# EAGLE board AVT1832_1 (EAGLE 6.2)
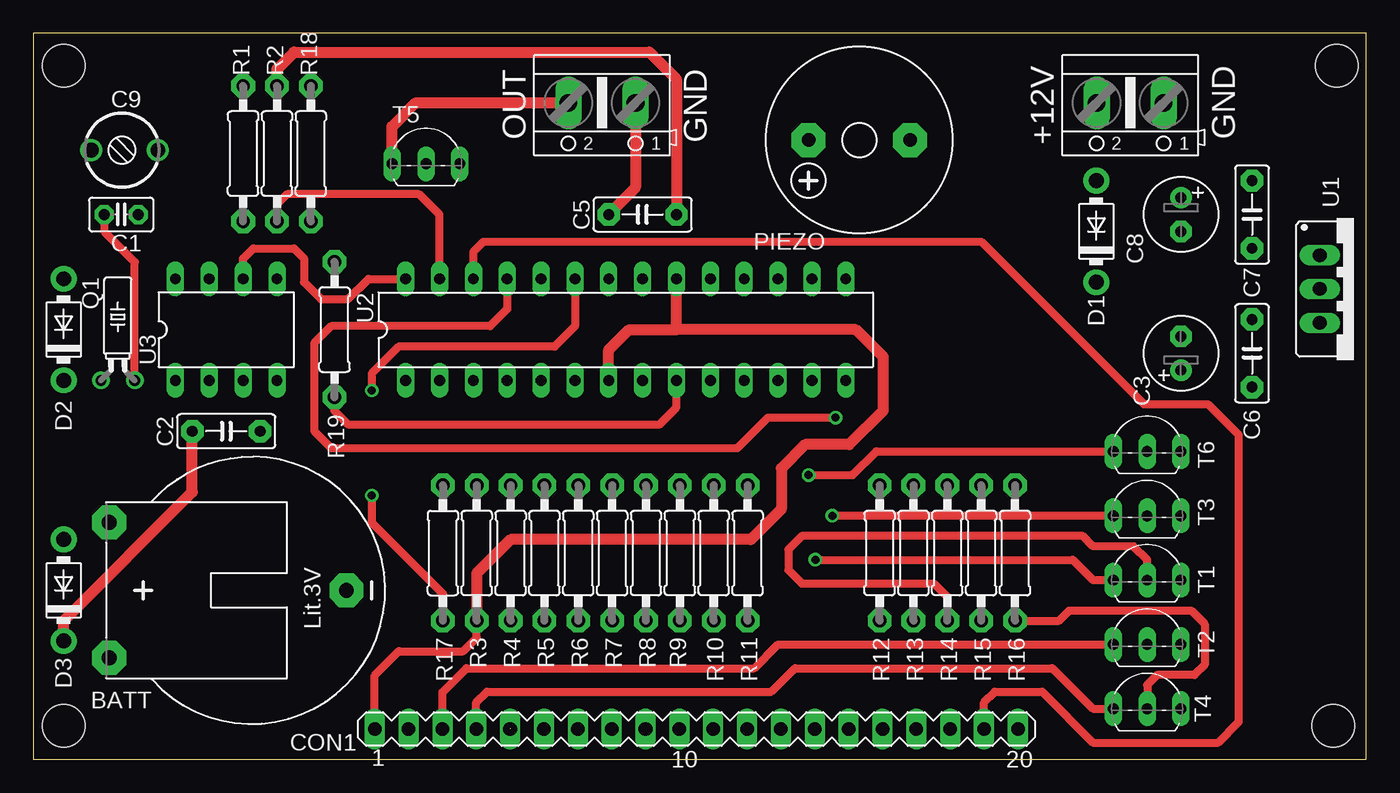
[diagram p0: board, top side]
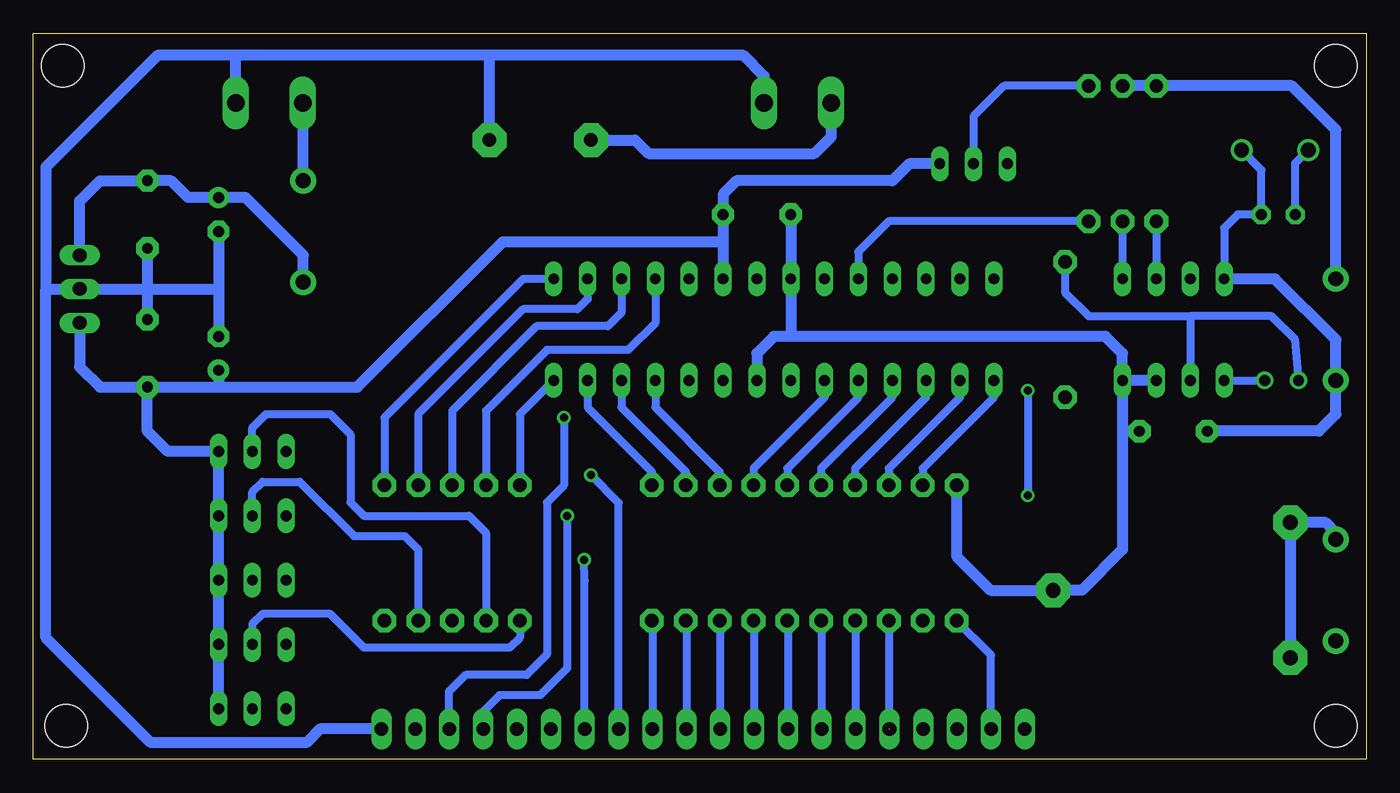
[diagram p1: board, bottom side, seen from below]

Size 99.99 x 54.49 mm. Coordinates in mm from the lower left corner, seen from the top.
Outline: 99.99,0 99.99,54.49 0,54.49 0,0 99.99,0
Copper layers (1*16): Top 0.035mm / dielectric 1.5mm / Bottom 0.035mm
Design rules: minimum track width 10mil, minimum drill 24mil, track to track 8mil, track to pad 8mil, pad to pad 8mil, via to via 8mil, smd to smd 8mil, copper to edge 40mil, drill to drill 8mil, minimum pad ring 10mil, minimum via ring 8mil, stop-mask expansion 4mil, vias tented up to drill 0mil, thermal gap 10mil
Holes 3.2 mm at 97.78,52.07 2.28,52.07 97.53,2.54 2.28,2.54

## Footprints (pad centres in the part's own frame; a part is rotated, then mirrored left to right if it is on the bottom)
AK500/2 = drill 1.321 long: 1 -2.515,0; 2 2.515,0
CR2032H = drill 1.118 pad 2.54 octagon: + 5.08,10.795; +@1 -5.08,10.795; - 0,-6.985
C025-025X050 = drill 0.813 pad 1.422 octagon: 1 -1.27,0; 2 1.27,0
C050-025X075 = drill 0.813 pad 1.676 octagon: 1 -2.54,0; 2 2.54,0
E2,5-6 = drill 0.813 pad 1.6: + -1.27,0 | drill 0.813 pad 1.6 octagon: - 1.27,0
CTRIM3050.504 = drill 1.1: 1 -2.5,0; 2 2.5,0
MA20-1 = drill 1.016 long: 1 -24.13,0; 2 -21.59,0; 3 -19.05,0; 4 -16.51,0; 5 -13.97,0; 6 -11.43,0; 7 -8.89,0; 8 -6.35,0; 9 -3.81,0; 10 -1.27,0; 11 1.27,0; 12 3.81,0; 13 6.35,0; 14 8.89,0; 15 11.43,0; 16 13.97,0; 17 16.51,0; 18 19.05,0; 19 21.59,0; 20 24.13,0
DO41-10 = drill 1.118 pad 1.93: A 3.81,0; C -3.81,0
F/CM12P = drill 1.016 pad 2.54 octagon: + 3.81,0; - -3.81,0
TC26H = drill 0.813: 1 -1.27,0; 2 1.27,0
0207/10 = drill 1 pad 1.778 octagon: 1 -5.08,0; 2 5.08,0
TO92-EBC = drill 0.813 long: B 0,-1.27; C -2.54,-1.27; E 2.54,-1.27
78XXS = drill 1.016 long: GND 0,-2.54; IN -2.54,-2.54; OUT 2.54,-2.54
DIL28-3 = drill 0.813 long: 1 -16.51,-3.81; 2 -13.97,-3.81; 3 -11.43,-3.81; 4 -8.89,-3.81; 5 -6.35,-3.81; 6 -3.81,-3.81; 7 -1.27,-3.81; 8 1.27,-3.81; 9 3.81,-3.81; 10 6.35,-3.81; 11 8.89,-3.81; 12 11.43,-3.81; 13 13.97,-3.81; 14 16.51,-3.81; 15 16.51,3.81; 16 13.97,3.81; 17 11.43,3.81; 18 8.89,3.81; 19 6.35,3.81; 20 3.81,3.81; 21 1.27,3.81; 22 -1.27,3.81; 23 -3.81,3.81; 24 -6.35,3.81; 25 -8.89,3.81; 26 -11.43,3.81; 27 -13.97,3.81; 28 -16.51,3.81
DIL08 = drill 0.813 long: 1 -3.81,-3.81; 2 -1.27,-3.81; 3 1.27,-3.81; 4 3.81,-3.81; 5 3.81,3.81; 6 1.27,3.81; 7 -1.27,3.81; 8 -3.81,3.81

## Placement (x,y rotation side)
+12V  [AK500/2]  82.29,49.28 180 top
BATT  CR2032H  [CR2032H]  16.5,12.7 90 top
C1  [C025-025X050]  6.59,40.89 0 top
C2  100nF  [C050-025X075]  14.47,24.64 0 top
C3  220uF  [E2,5-6]  86.1,30.48 90 top
C5  100nF  [C050-025X075]  45.71,40.89 180 top
C6  100nF  [C050-025X075]  91.43,30.48 90 top
C7  100nF  [C050-025X075]  91.43,40.89 270 top
C8  220uF  [E2,5-6]  86.1,40.89 270 top
C9  [CTRIM3050.504]  6.85,45.72 180 top
CON1  [MA20-1]  49.74,2.29 0 top
D1  1N4007  [DO41-10]  79.75,39.62 90 top
D2  1N4007  [DO41-10]  2.28,32.26 90 top
D3  1N4007  [DO41-10]  2.28,12.7 90 top
OUT  [AK500/2]  42.66,49.28 180 top
PIEZO  F/CM12P  [F/CM12P]  61.97,46.48 180 top
Q1  [TC26H]  6.34,28.45 0 top
R1  [0207/10]  15.74,45.47 90 top
R2  [0207/10]  18.28,45.47 90 top
R3  3,3k  [0207/10]  33.26,15.49 90 top
R4  [0207/10]  35.8,15.49 90 top
R5  [0207/10]  38.34,15.49 90 top
R6  [0207/10]  40.88,15.49 90 top
R7  [0207/10]  43.42,15.49 90 top
R8  [0207/10]  45.96,15.49 90 top
R9  [0207/10]  48.5,15.49 90 top
R10  [0207/10]  51.04,15.49 90 top
R11  [0207/10]  53.58,15.49 90 top
R12  [0207/10]  63.49,15.49 90 top
R13  47  [0207/10]  66.03,15.49 90 top
R14  [0207/10]  68.57,15.49 90 top
R15  [0207/10]  71.11,15.49 90 top
R16  [0207/10]  73.65,15.49 90 top
R17  [0207/10]  30.72,15.49 270 top
R18  [0207/10]  20.82,45.47 90 top
R19  [0207/10]  22.6,32.26 270 top
T1  [TO92-EBC]  83.56,14.73 0 top
T2  [TO92-EBC]  83.56,9.91 0 top
T3  [TO92-EBC]  83.56,19.56 0 top
T4  [TO92-EBC]  83.56,5.08 0 top
T5  [TO92-EBC]  29.45,45.97 0 top
T6  [TO92-EBC]  83.56,24.38 0 top
U1  7805  [78XXS]  99.05,35.31 270 top
U2  ATMEGA8  [DIL28-3]  44.44,32.26 0 top
U3  PFC8583P  [DIL08]  14.47,32.26 0 top

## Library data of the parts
+12V OUT = con-ptr500; OC_FARNELL: unknown; OC_NEWARK: unknown
BATT = battery
C1-C3 C5-C9 R1-R19 = rcl
CON1 = con-lstb; OC_FARNELL: unknown; OC_NEWARK: unknown
D1-D3 = diode
PIEZO = buzzer; OC_FARNELL: unknown; OC_NEWARK: unknown
Q1 = crystal; OC_FARNELL: unknown; OC_NEWARK: unknown
T1-T6 = transistor-pnp
U1 = v-reg
U2 = avr-4
U3 = micro-philips; OC_FARNELL: unknown; OC_NEWARK: unknown

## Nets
32K: R19.2 U2.9
+5V: C3.+ C5.1 C6.1 CON1.1 D2.A R1.2 R2.2 R3.1 T1.E T2.E T3.E T4.E T5.E T6.E U1.OUT U2.7 U2.20
+12V: C7.1 C8.+ D1.C U1.IN
A1: CON1.3 T2.C
A2: CON1.4 T4.C
A3: CON1.17 T3.C
A4: CON1.14 T1.C
A5: CON1.13 T6.C
GND: +12V.1 BATT.- C2.2 C3.- C5.2 C6.2 C7.2 C8.- CON1.20 OUT.1 PIEZO.- R17.1 U1.GND U2.8 U2.22 U3.3 U3.4
N$1: CON1.5 R4.1
N$2: CON1.6 R5.1
N$3: CON1.7 R6.1
N$4: CON1.8 R7.1
N$5: CON1.9 R8.1
N$6: CON1.10 R9.1
N$7: CON1.11 R10.1
N$8: CON1.12 R11.1
N$9: R18.2 T5.B
N$14: R14.1 T1.B
N$15: R12.1 T2.B
N$16: R15.1 T3.B
N$17: OUT.2 PIEZO.+ T5.C
N$18: R16.1 T4.B
N$19: R13.1 T6.B
N$22: BATT.+ D3.A
N$23: R3.2 U2.1
N$24: +12V.2 D1.A
N$25: C1.1 C9.2 Q1.2 U3.1
N$26: Q1.1 R19.1 U3.2
N$40: C1.2 C2.1 C9.1 D2.C D3.C U3.8
PIEZO: R18.1 U2.24
S1: CON1.18 U2.25
S2: CON1.19 U2.26
SA: R4.2 U2.2
SB: R5.2 U2.3
SC: R6.2 U2.4
SCL: R1.1 U2.28 U3.6
SD: R7.2 U2.5
SDA: R2.1 U2.27 U3.5
SDP: R11.2 U2.13
SE: R8.2 U2.6
SF: R9.2 U2.11
SG: R10.2 U2.12
TA1: R12.2 U2.14
TA2: R16.2 U2.15
TA3: R15.2 U2.16
TA4: R14.2 U2.17
TA5: R13.2 U2.18
TERM: CON1.2 R17.2 U2.23

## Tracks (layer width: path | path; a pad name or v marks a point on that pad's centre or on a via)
32K
  Top 0.61: R19.2 22.6,26.16 23.61,25.15 46.98,25.15 48.25,26.42 U2.9
+5V
  Top 0.61: CON1.1 25.61,6.31 27.42,8.13 32.25,8.13 33.26,9.14 R3.1 | U2.20 48.25,35.05
  Top 0.813: R3.1 33.26,13.97 35.8,16.51 53.84,16.51 56.12,18.8 56.12,21.84 57.9,23.62 61.2,23.62 63.74,26.16 63.74,30.23 61.71,32.26 48.25,32.26 | 48.25,32.26 U2.20 | R2.2 18.28,51.82 19.55,53.09 46.22,53.09 48.25,51.05 C5.1 | U2.7 43.17,30.73 44.69,32.26 48.25,32.26
  Bottom 0.61: 91.43,27.69 91.18,27.94 C6.1
  Bottom 0.813: R2.2 R1.2 5.58,50.55 2.28,47.24 D2.A | 48.25,38.86 C5.1 48.25,42.42 47.23,43.43 35.55,43.43 34.28,44.7 T5.E | 48.25,38.86 U2.20 | T4.E T2.E T1.E T3.E T6.E 89.91,23.11 91.43,24.64 91.43,27.69 | 86.1,27.94 C6.1 94.99,27.94 96.51,29.46 U1.OUT | C3.+ 86.1,27.94 | 86.1,27.94 75.68,27.94 64.76,38.86 48.25,38.86
+12V
  Bottom 0.813: U1.IN 96.51,41.91 94.99,43.43 C7.1 89.65,43.43 88.38,42.16 C8.+ 84.06,42.16 79.75,37.85 D1.C
A1
  Top 0.61: CON1.3 30.69,5.04 32.5,6.86 54.09,6.86 55.87,8.64 T2.C
A2
  Top 0.61: CON1.4 33.23,4.28 34.03,5.08 55.36,5.08 57.14,6.86 76.44,6.86 79.49,3.81 T4.C
A3  (via drill 0.6)
  Top 0.61: T3.C v59.93,18.29
  Bottom 0.61: v59.93,18.29 59.93,6.86 61.97,4.83 65.01,4.83 66.28,3.56 66.28,2.32 CON1.17
A4  (via drill 0.6)
  Top 0.61: v58.66,14.99 77.97,14.99 79.49,13.46 T1.C
  Bottom 0.61: CON1.14 58.63,13.42 v58.66,14.99
A5  (via drill 0.6)
  Top 0.61: v58.16,21.34 61.46,21.34 63.24,23.11 T6.C
  Bottom 0.61: CON1.13 56.09,19.27 v58.16,21.34
GND
  Top 0.813: OUT.1 45.18,42.9 C5.2
  Bottom 0.813: U3.4 18.28,24.64 | 18.28,24.64 18.28,15.75 21.33,12.7 BATT.- 28.18,12.7 30.72,15.24 R17.1 | C2.2 18.28,24.64 | U3.3 U3.4 | 43.17,31.75 U2.22 C5.2 | U2.8 45.71,30.48 44.44,31.75 43.17,31.75 | U3.4 18.28,30.48 19.55,31.75 43.17,31.75 | PIEZO.- 65.78,52.83 | 65.78,52.83 84.57,52.83 | 84.57,52.83 90.67,52.83 99.05,44.45 99.05,35.31 | 99.05,35.31 U1.GND 91.43,35.31 | C7.2 91.43,35.31 | 91.43,35.31 C6.2 | C8.- 86.1,35.31 | 86.1,35.31 C3.- | 91.43,35.31 86.1,35.31 | +12V.1 84.8,52.6 84.57,52.83 | OUT.1 45.18,51.28 46.73,52.83 65.78,52.83 | CON1.20 78.48,2.29 79.49,1.27 91.18,1.27 99.05,9.14 99.05,35.31
N$1  (1 unrouted)
  Bottom 0.61: R4.1 35.8,2.29
N$2
  Bottom 0.61: R5.1 38.31,10.41 CON1.6
N$3
  Bottom 0.61: R6.1 40.85,10.41 CON1.7
N$4
  Bottom 0.61: R7.1 43.39,10.41 CON1.8
N$5
  Bottom 0.61: R8.1 45.93,10.41 CON1.9
N$6
  Bottom 0.61: R9.1 48.47,10.41 CON1.10
N$7
  Bottom 0.61: R10.1 51.01,10.41 CON1.11
N$8
  Bottom 0.61: R11.1 53.55,10.41 CON1.12
N$9
  Bottom 0.61: R18.2 27.17,50.55 29.45,48.26 T5.B
N$10
  Bottom 0.813: 5.71,17.78 5.71,7.62
N$14
  Top 0.61: T1.B 83.56,14.99 82.54,16 79.49,16 78.73,16.76 57.65,16.76 56.63,15.75 56.63,14.22 57.65,13.21 67.55,13.21 68.57,12.19 R14.1
N$15
  Bottom 0.61: R12.1 63.49,9.14 64.25,8.38 75.17,8.38 77.71,10.92 82.79,10.92 83.56,10.16 T2.B
N$16
  Bottom 0.61: T3.B 83.56,20.07 82.79,20.83 80,20.83 75.94,16.76 72.13,16.76 71.11,15.75 R15.1
N$17
  Top 0.813: T5.C 26.91,47.5 28.69,49.28 OUT.2
  Bottom 0.813: PIEZO.+ 54.85,46.48 53.84,45.47 41.39,45.47 40.12,46.74 40.12,49.25 OUT.2
N$18
  Top 0.61: R16.1 76.95,10.41 77.71,11.18 86.86,11.18 87.87,10.16 87.87,7.11 87.11,6.35 84.32,6.35 83.56,5.59 T4.B
N$19
  Bottom 0.61: T6.B 83.56,24.89 82.54,25.91 77.71,25.91 76.19,24.38 76.19,19.3 75.17,18.29 67.3,18.29 66.03,17.02 R13.1
N$22
  Bottom 0.813: D3.A 2.28,17.02 3.04,17.78 BATT.+
N$23
  Bottom 0.61: U2.1 27.93,27.18 33.26,21.84 R3.2
N$24
  Bottom 0.813: +12V.2 79.77,43.46 D1.A
N$25
  Top 0.61: Q1.2 7.61,37.34 5.32,39.62 C1.1
  Bottom 0.61: U3.1 Q1.2 | C1.1 5.32,44.74 C9.2
N$26
  Bottom 0.61: Q1.1 5.32,31.5 7.1,33.27 13.2,33.27 | 13.2,33.27 U3.2 | R19.1 22.6,35.05 20.82,33.27 13.2,33.27
N$40
  Top 0.813: C2.1 11.93,20.07 2.28,10.41 D3.C
  Bottom 0.61: C9.1 7.86,44.24 C1.2 9.64,40.89 10.66,39.88 U3.8
  Bottom 0.813: C2.1 3.55,24.64 2.28,25.91 D2.C 2.28,31.5 6.85,36.07 U3.8
PIEZO
  Bottom 0.61: R18.1 35.8,40.39 38.09,38.1 U2.24
S1  (via drill 0.6)
  Top 0.61: U2.25 35.55,33.78 34.28,32.51 22.34,32.51 21.07,31.24 21.07,24.64 22.34,23.37 52.82,23.37 55.11,25.65 v60.19,25.65
  Bottom 0.61: v60.19,25.65 60.19,20.57 61.46,19.3 61.46,7.87 62.98,6.35 67.55,6.35 68.82,5.08 68.82,2.32 CON1.18
S2
  Top 0.61: U2.26 33.01,38.1 33.77,38.86 71.11,38.86 83.3,26.67 88.13,26.67 90.41,24.38 90.41,2.79 88.89,1.27 79.49,1.27 75.68,5.08 72.13,5.08 71.33,4.28 CON1.19
SA
  Bottom 0.61: U2.2 30.47,27.18 35.8,21.84 R4.2
SB
  Bottom 0.61: U2.3 33.01,27.18 38.34,21.84 R5.2
SC
  Bottom 0.61: U2.4 35.55,27.18 40.88,21.84 R6.2
SCL
  Top 0.61: U3.6 15.74,37.59 16.5,38.35 19.55,38.35 20.31,37.59 20.31,35.81 21.58,34.54 23.61,34.54 25.14,36.07 U2.28
  Bottom 0.61: R1.1 U3.6
SD
  Bottom 0.61: U2.5 38.09,27.18 43.42,21.84 R7.2
SDA
  Top 0.61: U2.27 30.47,40.89 28.95,42.42 19.04,42.42 18.28,41.66 R2.1
  Bottom 0.61: R2.1 U3.5
SDP
  Bottom 0.61: U2.13 58.41,26.42 53.58,21.59 R11.2
SE
  Bottom 0.61: U2.6 40.63,27.18 45.96,21.84 R8.2
SF
  Bottom 0.61: U2.11 53.33,26.42 48.5,21.59 R9.2
SG
  Bottom 0.61: U2.12 55.87,26.42 51.04,21.59 R10.2
TA1
  Bottom 0.61: U2.14 63.49,25.91 R12.2 63.49,20.32
TA2
  Bottom 0.61: U2.15 63.24,36.07 73.65,25.65 R16.2
TA3
  Bottom 0.61: U2.16 58.41,34.54 59.17,33.78 63.24,33.78 71.11,25.91 R15.2
TA4
  Bottom 0.61: U2.17 55.87,33.53 56.89,32.51 62.22,32.51 68.57,26.16 R14.2
TA5
  Bottom 0.61: U2.18 53.33,32.77 55.36,30.73 61.46,30.73 66.03,26.16 R13.2
TERM  (via drill 0.6)
  Top 0.61: U2.23 40.63,32.51 39.11,30.99 27.42,30.99 25.39,28.96 v25.39,27.69 | v25.39,19.81 25.39,17.78 30.72,12.45 R17.2
  Bottom 0.61: CON1.2 28.15,7.84 R17.2 | v25.39,27.69 v25.39,19.81

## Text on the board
tNames: GND | GND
